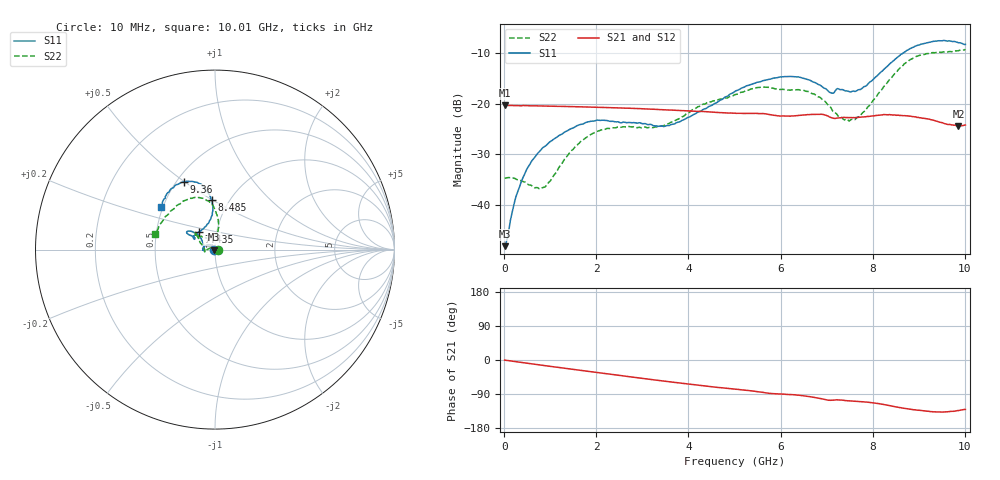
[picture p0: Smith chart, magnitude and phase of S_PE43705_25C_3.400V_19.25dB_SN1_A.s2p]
! Device ID: PE43705
! Serial: 1
! Insertion: A
! Impedance: 50 ohm
! Temp: 25C
! VDD: 3.400V
! Attenuation Step: 19.25dB
#  Hz  S  RI  R  50
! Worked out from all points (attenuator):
!   401 points, 10 MHz to 10.01 GHz, reference 50 ohm
!   highest |S21| = -20.32 dB at 10 MHz (marker M1); lowest = -24.4 dB at 9.86 GHz (marker M2)
!   lowest |S11| = -48.1 dB at 10 MHz (marker M3), VSWR 1.01, Z = 49.6 + j0.0425 ohm
!   |S11| at or under -10 dB: start of sweep to 8.66 GHz
!   |S22| runs from -36.8 to -9.3 dB; largest |S21 - S12| = 0.0011
!   S11 on the Smith chart (normalised r, x): 10 MHz: 0.99, +0.00; 7.435 GHz: 0.82, +0.16; 8.485 GHz: 0.83, +0.49; 9.36 GHz: 0.55, +0.50; 10.01 GHz: 0.49, +0.27
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1e7  -0.0039 0.000428  0.0964 -0.000417  0.0965 -0.000398  0.0183 0.000218
2.85e8  -0.00567 0.0119  0.0954 -0.00817  0.0955 -0.00808  0.0161 0.00754
5.6e8  -0.0128 0.0219  0.0941 -0.0158  0.0941 -0.0157  0.00882 0.013
9.1e8  -0.0278 0.0269  0.0915 -0.025  0.0916 -0.0249  -0.00666 0.014
1.685e9  -0.0604 0.0169  0.0824 -0.0433  0.0824 -0.0433  -0.0431 0.000677
2.235e9  -0.0683 0.00118  0.0736 -0.0545  0.0737 -0.0544  -0.056 -0.0111
3.36e9  -0.0598 0.00365  0.0515 -0.071  0.0515 -0.0709  -0.0591 0.00283
3.86e9  -0.0631 0.0266  0.0409 -0.0751  0.0409 -0.0748  -0.0706 0.0231
4.385e9  -0.0729 0.0525  0.0301 -0.0778  0.0302 -0.0777  -0.0872 0.0508
5.01e9  -0.1 0.0868  0.0182 -0.0784  0.0183 -0.0785  -0.0983 0.0741
5.56e9  -0.1304 0.1006  0.00759 -0.0796  0.00762 -0.0796  -0.1119 0.093
6.01e9  -0.1531 0.1017  0.000256 -0.0755  0.00067 -0.0759  -0.1055 0.0895
6.685e9  -0.1439 0.0821  -0.0108 -0.0776  -0.0107 -0.0774  -0.0988 0.0779
7.085e9  -0.1105 0.0655  -0.0206 -0.0704  -0.0208 -0.0706  -0.0589 0.071
7.435e9  -0.0917 0.0973  -0.0218 -0.0697  -0.0215 -0.0696  -0.0216 0.0671
7.76e9  -0.0483 0.1324  -0.0254 -0.0695  -0.0252 -0.0693  0.00504 0.0796
8.36e9  -0.0118 0.2452  -0.0393 -0.0675  -0.0394 -0.0673  0.0161 0.1716
8.485e9  -0.0181 0.275  -0.0425 -0.0649  -0.0421 -0.065  0.00821 0.2002
8.885e9  -0.0698 0.3549  -0.0491 -0.0561  -0.0485 -0.0565  -0.0515 0.2784
9.36e9  -0.1715 0.3767  -0.0496 -0.0462  -0.0494 -0.0463  -0.1616 0.2752
9.86e9  -0.2773 0.2869  -0.0415 -0.0437  -0.0416 -0.0436  -0.2972 0.152
1.001e10  -0.3011 0.24  -0.04 -0.047  -0.0401 -0.0473  -0.3328 0.0877
